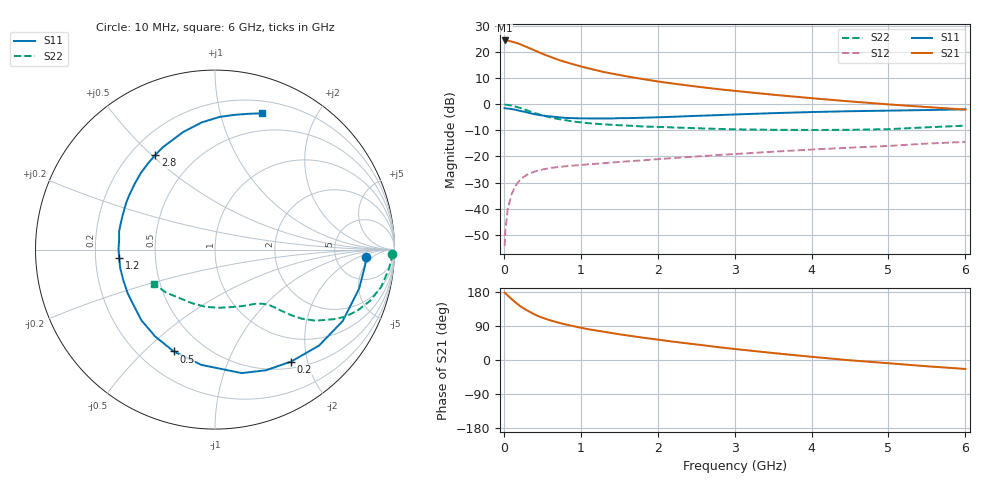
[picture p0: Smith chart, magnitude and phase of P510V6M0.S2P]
! SIEMENS Small Signal Semiconductors
! BFP183
! Si NPN RF Bipolar Junction Transistor in SOT143
! VCE = 10 V  IC = 6 mA
! Common Emitter S-Parameters:  March  1996
# GHz  S  MA  R  50
!  f  S11  S21  S12  S22
! GHz  MAG  ANG  MAG  ANG  MAG  ANG  MAG  ANG
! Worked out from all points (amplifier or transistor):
!   36 points, 10 MHz to 6 GHz, reference 50 ohm
!   highest |S21| = 24.5 dB at 10 MHz (marker M1)
!   |S21| within 3 dB of that: start of sweep to 336.1 MHz
!   unconditionally stable (mu >= 1): 1.588 GHz to 5.842 GHz
!   at 250 MHz: K = 0.22, MSG = 25.3 dB, |S12| = -28.0 dB
!   at 1.4 GHz: K = 0.94, MSG = 17.1 dB, |S12| = -22.3 dB
!   at 6 GHz: K = 0.98, MSG = 6.2 dB, |S12| = -14.4 dB
!   S11 on the Smith chart (normalised r, x): 10 MHz: 11, -3; 200 MHz: 0.60, -1.73; 500 MHz: 0.34, -0.62; 1.2 GHz: 0.30, -0.04; 2.8 GHz: 0.30, +0.51; 6 GHz: 0.32, +1.35
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0.01  0.8432 -2.9  16.86 177.7  0.0019 81.7  0.9867 -1.3
0.02  0.8407 -6.1  16.71 176.3  0.0038 84.5  0.9858 -2.6
0.05  0.832 -15.1  16.73 170.3  0.0097 84.2  0.9751 -6.4
0.1  0.8153 -29.2  16.06 161.1  0.0188 73.4  0.9485 -12.7
0.15  0.7886 -42.7  15.32 152.3  0.0272 67.6  0.9099 -18.3
0.2  0.7544 -55.8  14.55 144.2  0.0339 62.6  0.8641 -23.1
0.25  0.7298 -67.1  13.47 137.2  0.0399 57.7  0.8156 -27.3
0.3  0.7039 -77.8  12.58 131.2  0.0445 52.9  0.7685 -30.3
0.4  0.6469 -96.7  10.89 120.1  0.0514 46.8  0.6851 -35.3
0.5  0.6122 -112.0  9.369 111.6  0.0561 41.5  0.6162 -38.6
0.6  0.588 -124.4  8.229 104.9  0.0601 38.6  0.5658 -40.5
0.7  0.5688 -136.0  7.238 99.1  0.0626 36.8  0.5267 -41.8
0.9  0.5441 -153.4  5.906 89.5  0.067 34.2  0.4711 -43.7
1.1  0.5379 -169.0  4.924 81.1  0.0708 33.4  0.4355 -45.4
1.2  0.5364 -174.8  4.525 77.9  0.0726 32.9  0.4242 -46.3
1.6  0.5451 164.5  3.45 65.0  0.0805 32.8  0.3921 -50.3
2.2  0.5781 140.8  2.512 48.4  0.0932 33.0  0.3608 -58.9
2.8  0.6235 122.2  1.952 33.6  0.1071 32.2  0.3386 -70.1
3.5  0.6786 105.2  1.533 18.4  0.1236 30.2  0.3249 -85.6
4.5  0.7399 88.0  1.139 -0.8  0.1477 25.5  0.325 -113.2
5.5  0.7791 76.2  0.89 -16.6  0.1768 20.5  0.3631 -138.8
6  0.8032 71.0  0.794 -23.6  0.1906 16.7  0.3904 -150.8
